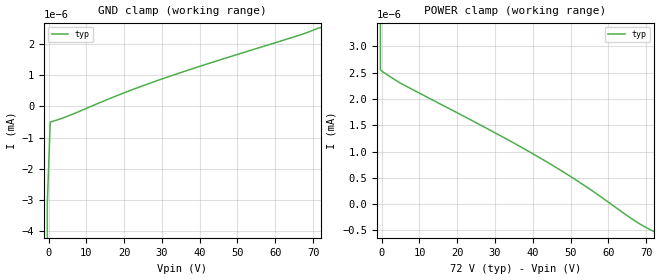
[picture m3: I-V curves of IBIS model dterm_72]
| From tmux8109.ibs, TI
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| dterm_72
[Model]   dterm_72
Model_type   Terminator
|   typ   min   max
C_comp   4.014581e-12   NA   NA
[Voltage Range]   72   NA   NA
[Temperature Range]   27   NA   NA
[Power Clamp Reference]   72   NA   NA
[GND Clamp Reference]   0   NA   NA
[GND Clamp]
|   Voltage   I(typ)   I(min)   I(max)
-5V       -2.258A    NA         NA
-1.111V   -40.05mA   NA         NA
-333.3mV  -3.131nA   NA         NA
444.4mV   -505.4pA   NA         NA
5.111V    -313.9pA   NA         NA
18.33V    352.5pA    NA         NA
29.22V    841.9pA    NA         NA
42.44V    1.374nA    NA         NA
66.56V    2.284nA    NA         NA
72V       2.519nA    NA         NA
[POWER Clamp]
|   Voltage   I(typ)   I(min)   I(max)
-5V       744mA      NA         NA
-1.111V   26.13mA    NA         NA
-333.3mV  2.556nA    NA         NA
444.4mV   2.508nA    NA         NA
5.111V    2.297nA    NA         NA
29.22V    1.387nA    NA         NA
42.44V    856pA      NA         NA
53.33V    368.5pA    NA         NA
67.33V    -334.5pA   NA         NA
72V       -522.1pA   NA         NA
